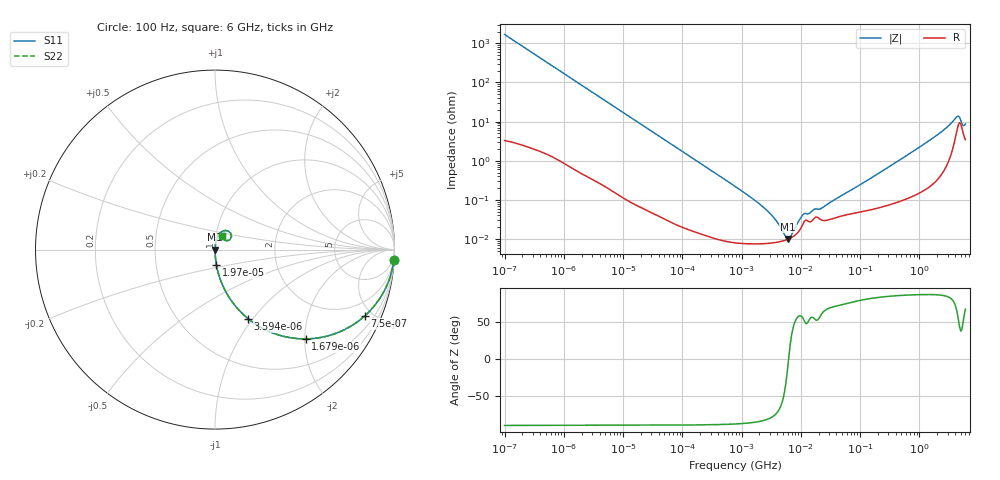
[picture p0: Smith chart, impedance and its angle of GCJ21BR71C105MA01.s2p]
!Murata Part Number: GCJ21BR71C105MA01
!These Parameters are Measured in Series Mode Connection
!Data Generated on Mar 13, 2026
!  o--ll--o
!Port1  Port2
!  o------o
!Operation Temp=25[degC], DC Bias Voltage=0[V]
!Freq. Start=100[Hz] Stop=6[GHz] 401[Steps]
# Hz S RI R 50
!Freq.(Hz) S11(Real) S11(Imag) S21(Real) S21(Imag) S12(Real) S12(Imag) S22(Real) S22(Imag)
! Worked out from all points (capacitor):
!   401 points, 100 Hz to 6 GHz, reference 50 ohm
!   read as one part in series: C = 942 nF near 109 Hz
!   lowest |Z| = 9.98 mohm at 6.075 MHz (marker M1)
!   series resonance near 6.225 MHz, so ESL is about 690 pH
!   S11 on the Smith chart (normalised r, x): 100 Hz: 1, -34; 750 Hz: 1.02, -4.52; 1.679 kHz: 1.01, -2.03; 3.594 kHz: 1.01, -0.95; 19.7 kHz: 1.00, -0.17; 6 GHz: 1.07, +0.16
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100  0.9964 -0.059  0.00361 0.059  0.00361 0.059  0.9964 -0.059
350  0.9582 -0.1983  0.0418 0.1983  0.0418 0.1983  0.9582 -0.1983
750  0.8352 -0.3686  0.1648 0.3686  0.1648 0.3686  0.8352 -0.3686
1679  0.5062 -0.4973  0.4938 0.4973  0.4938 0.4973  0.5062 -0.4973
2008  0.4182 -0.4905  0.5818 0.4905  0.5818 0.4905  0.4182 -0.4905
3594  0.1851 -0.3854  0.8149 0.3854  0.8149 0.3854  0.1851 -0.3854
7036  0.0571 -0.2288  0.9429 0.2288  0.9429 0.2288  0.0571 -0.2288
19704  0.00816 -0.0863  0.9918 0.0863  0.9918 0.0863  0.00816 -0.0863
40335  0.0022 -0.0426  0.9978 0.0426  0.9978 0.0426  0.0022 -0.0426
774597  8.47e-05 -0.00222  0.9999 0.00222  0.9999 0.00222  8.47e-05 -0.00222
2837864  7.76e-05 -0.00049  0.9999 0.00049  0.9999 0.00049  7.76e-05 -0.00049
3882480  8.22e-05 -0.000277  0.9999 0.000277  0.9999 0.000277  8.22e-05 -0.000277
5554849  9.39e-05 -6.51e-05  0.9999 6.51e-05  0.9999 6.51e-05  9.39e-05 -6.51e-05
6075234  9.88e-05 -1.39e-05  0.9999 1.39e-05  0.9999 1.39e-05  9.88e-05 -1.39e-05
6948629  0.000109 6.4e-05  0.9999 -6.4e-05  0.9999 -6.4e-05  0.000109 6.4e-05
1.039699e7  0.00021 0.00032  0.9998 -0.00032  0.9998 -0.00032  0.00021 0.00032
1.555665e7  0.000295 0.000433  0.9997 -0.000433  0.9997 -0.000433  0.000295 0.000433
2.327686e7  0.0003 0.000557  0.9997 -0.000557  0.9997 -0.000557  0.0003 0.000557
3.124326e8  0.000794 0.00705  0.9992 -0.00705  0.9992 -0.00705  0.000794 0.00705
1.873145e9  0.00466 0.0419  0.9953 -0.0419  0.9953 -0.0419  0.00466 0.0419
4.193612e9  0.0578 0.1067  0.9422 -0.1067  0.9422 -0.1067  0.0578 0.1067
6e9  0.0392 0.0745  0.9608 -0.0745  0.9608 -0.0745  0.0392 0.0745
